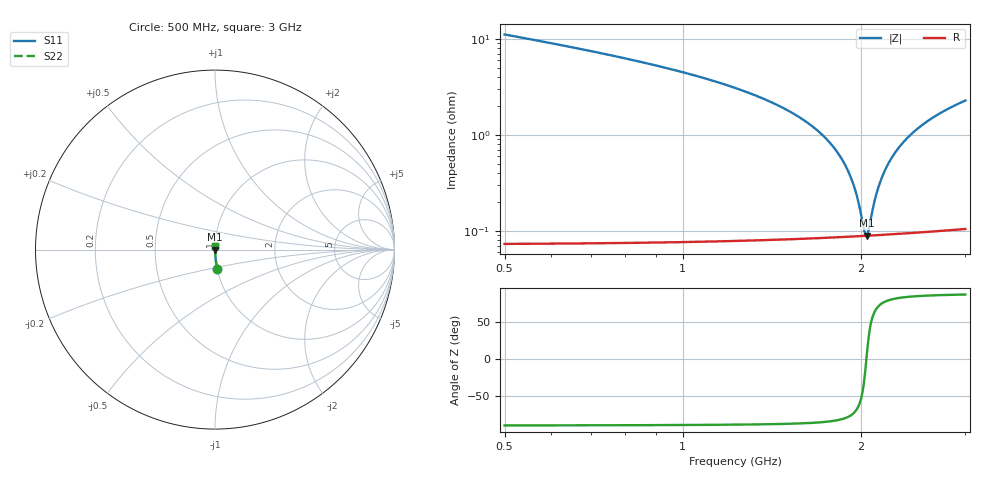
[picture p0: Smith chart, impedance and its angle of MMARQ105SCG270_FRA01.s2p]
! MMARQ105SCG270_FRA01  S-PARAMETER MODEL  ( General Type )
! Model Generated by TAIYO YUDEN Corporation (http://www.ty-top.com)
! Version 1.0
! TAIYO YUDEN Control No. 200326
! Copyright(c) 2020 TAIYO YUDEN CO.,LTD. All Rights Reserved.
! Product Description (link to TY-COMPAS)
! https://ds.yuden.co.jp/TYCOMPAS/or/detail?pn=MMARQ105SCG270JFRA01&u=M
! Products Name : Multilayer Ceramic Capacitors
! Characteristics :
!  Capacitance : 27 pF , Rated Voltage : 250V , TCC : CG / C0G
!  Case Size : 1.0 x 0.5 / 0.039 x 0.02 [mm/inch] , Thickness : 0.5 / 0.02 [mm/inch]
!  (Conditions: Temperature = 25 degC , DC Bias Current/Voltage = 0A / 0V)
! External Node Assignments :
!  1  o---| |---o  2
! GND o---------o GND
! Frequency Range : 500MHz  -  3GHz  [ 401 STEP ]
# MHz S RI R 50
! Freq[MHz].  S11 Real  S11 Imag  S21 Real  S21 Imag  S12 Real  S12 Imag  S22 Real  S22 Imag
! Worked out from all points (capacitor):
!   401 points, 500 MHz to 3 GHz, reference 50 ohm
!   read as one part in series: C = 27 pF near 512.5 MHz
!   lowest |Z| = 89 mohm at 2.044 GHz (marker M1)
!   series resonance near 2.041 GHz, so ESL is about 230 pH
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500  0.0128 -0.1093  0.9872 0.1093  0.9872 0.1093  0.0128 -0.1093
918.75  0.00336 -0.0509  0.9966 0.0509  0.9966 0.0509  0.00336 -0.0509
1337.5  0.00142 -0.0251  0.9986 0.0251  0.9986 0.0251  0.00142 -0.0251
1575  0.00105 -0.0151  0.9989 0.0151  0.9989 0.0151  0.00105 -0.0151
1750  0.000924 -0.0089  0.9991 0.0089  0.9991 0.0089  0.000924 -0.0089
1843.75  0.000892 -0.00587  0.9991 0.00587  0.9991 0.00587  0.000892 -0.00587
1912.5  0.000882 -0.00376  0.9991 0.00376  0.9991 0.00376  0.000882 -0.00376
1943.75  0.00088 -0.00282  0.9991 0.00282  0.9991 0.00282  0.00088 -0.00282
1968.75  0.00088 -0.00209  0.9991 0.00209  0.9991 0.00209  0.00088 -0.00209
2025  0.000884 -0.000463  0.9991 0.000463  0.9991 0.000463  0.000884 -0.000463
2037.5  0.000886 -0.000109  0.9991 0.000109  0.9991 0.000109  0.000886 -0.000109
2043.75  0.000887 6.7e-05  0.9991 -6.7e-05  0.9991 -6.7e-05  0.000887 6.7e-05
2062.5  0.00089 0.000593  0.9991 -0.000593  0.9991 -0.000593  0.00089 0.000593
2093.75  0.000896 0.00146  0.9991 -0.00146  0.9991 -0.00146  0.000896 0.00146
2118.75  0.000902 0.00214  0.9991 -0.00214  0.9991 -0.00214  0.000902 0.00214
2168.75  0.000918 0.00348  0.9991 -0.00348  0.9991 -0.00348  0.000918 0.00348
2237.5  0.000944 0.00529  0.9991 -0.00529  0.9991 -0.00529  0.000944 0.00529
2331.25  0.00099 0.00766  0.999 -0.00766  0.999 -0.00766  0.00099 0.00766
2443.75  0.00106 0.0104  0.9989 -0.0104  0.9989 -0.0104  0.00106 0.0104
2587.5  0.00116 0.0138  0.9988 -0.0138  0.9988 -0.0138  0.00116 0.0138
2781.25  0.00133 0.0181  0.9987 -0.0181  0.9987 -0.0181  0.00133 0.0181
3000  0.00156 0.0227  0.9984 -0.0227  0.9984 -0.0227  0.00156 0.0227
